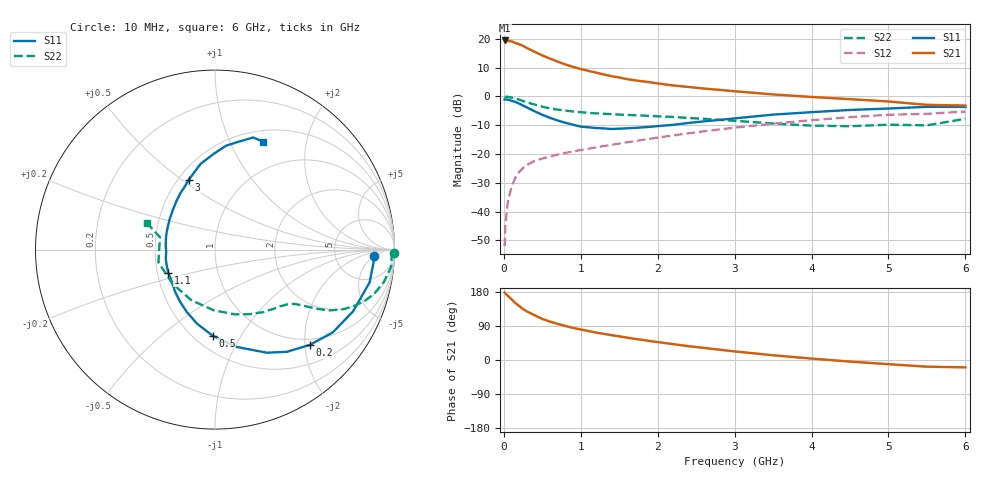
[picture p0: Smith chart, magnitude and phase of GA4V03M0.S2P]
! Infineon Technologies  Discrete & RF Semiconductors
! BF775
! Si NPN RF Bipolar Junction Transistor in SOT23
! VCE = 4 V  IC = 3 mA
! Common Emitter S-Parameters:  May  1996
# GHz  S  MA  R  50
!  f  S11  S21  S12  S22
! GHz  MAG  ANG  MAG  ANG  MAG  ANG  MAG  ANG
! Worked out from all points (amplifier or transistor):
!   36 points, 10 MHz to 6 GHz, reference 50 ohm
!   highest |S21| = 19.5 dB at 10 MHz (marker M1)
!   |S21| within 3 dB of that: start of sweep to 328.3 MHz
!   unconditionally stable (mu >= 1): 992.9 MHz to 3.486 GHz
!   at 250 MHz: K = 0.36, MSG = 21.2 dB, |S12| = -24.9 dB
!   at 1.4 GHz: K = 1.12, MAG = 9.8 dB, |S12| = -16.8 dB
!   at 6 GHz: K = 0.97, MSG = 1.0 dB, |S12| = -5.2 dB
!   S11 on the Smith chart (normalised r, x): 10 MHz: 15, -5; 200 MHz: 0.87, -2.11; 500 MHz: 0.61, -0.76; 1.1 GHz: 0.57, -0.16; 3 GHz: 0.56, +0.53; 6 GHz: 0.63, +1.34
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0.01  0.8861 -2.4  9.398 178.0  0.0025 87.8  0.9961 -1.0
0.02  0.8859 -4.9  9.281 175.8  0.0058 83.3  0.9846 -2.3
0.05  0.8806 -12.0  9.215 169.9  0.0141 82.7  0.9864 -5.5
0.1  0.8427 -24.1  9.083 160.2  0.027 76.5  0.958 -10.8
0.15  0.8023 -35.1  8.502 150.4  0.0389 71.0  0.9213 -15.4
0.2  0.7492 -45.1  8.073 142.3  0.0486 66.5  0.8803 -19.1
0.25  0.696 -54.9  7.557 134.5  0.0572 62.0  0.8321 -22.3
0.3  0.6431 -63.3  6.945 128.2  0.0643 59.5  0.7908 -24.8
0.4  0.5529 -78.1  5.967 118.0  0.076 54.9  0.7218 -28.0
0.5  0.4799 -91.6  5.155 108.5  0.0834 52.3  0.6641 -29.9
0.6  0.424 -103.8  4.546 101.4  0.0906 50.9  0.6197 -31.2
0.7  0.382 -114.1  4.028 95.3  0.0978 50.5  0.5901 -32.2
0.8  0.349 -124.1  3.597 89.8  0.1043 50.2  0.5674 -33.0
0.9  0.3227 -133.7  3.258 84.8  0.1111 50.2  0.5483 -33.8
1.1  0.2909 -153.6  2.783 76.5  0.1234 51.0  0.5188 -35.7
1.6  0.2794 168.6  2.004 59.1  0.1596 52.1  0.4777 -41.9
2.2  0.3211 137.3  1.55 41.9  0.2098 51.2  0.44 -52.4
3  0.4154 110.6  1.231 22.7  0.2868 46.0  0.3776 -72.9
3.5  0.4833 99.7  1.084 12.5  0.3359 41.0  0.3381 -91.3
4.5  0.5825 83.9  0.897 -4.2  0.4372 28.7  0.3038 -141.7
5.5  0.6597 71.2  0.715 -17.7  0.4988 13.2  0.3147 167.3
6  0.6589 65.9  0.694 -19.4  0.5466 8.8  0.409 158.5
